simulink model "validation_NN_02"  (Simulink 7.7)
settings: Solver=VariableStepDiscrete  StartTime=0.0  StopTime=100  RelTol=1e-3
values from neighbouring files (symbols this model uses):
  A = [0.9944 -0.1203 -0.4302    [process_model02.m]
  B = [1 0    [process_model02.m]
  C = [1 0 0    [process_model02.m]
  D = zeros(2,2)    [process_model02.m]
  Ts = 0.1    [process_model02.m]
  x0 = [0.01 0.02 0.03]    [process_model02.m]
libraries: neural x21, simulink x6

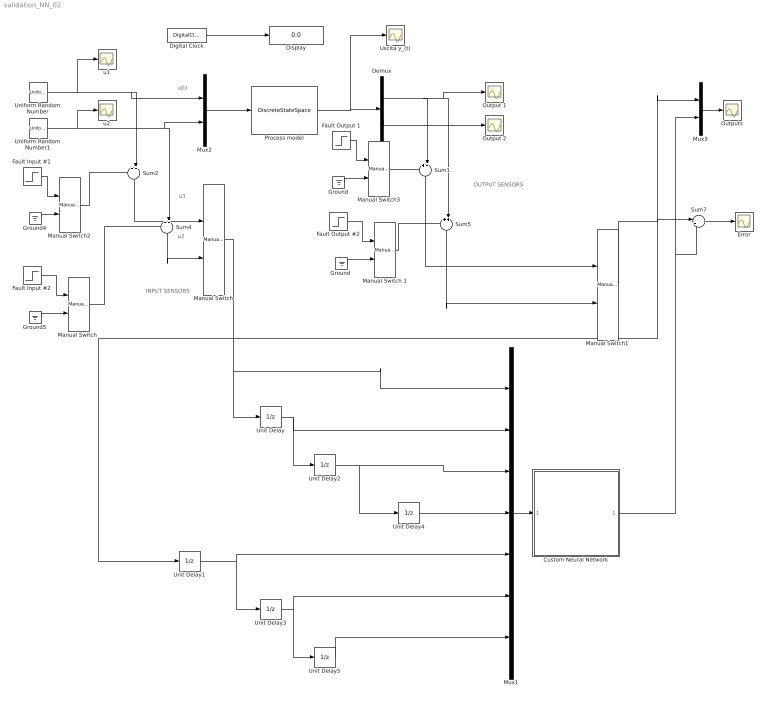
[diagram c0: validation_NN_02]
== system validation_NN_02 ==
  note: u(t)
  note: INPUT SENSORS
  note: OUTPUT SENSORS
  note: u1
  note: u2
  Custom Neural Network : Subsystem
  Demux : Demux  Outputs=2
  Digital Clock : DigitalClock  SampleTime=Ts
  Display : Display
  Error : Scope
  Fault Input #1 : Step  Time=50  After=5  SampleTime=Ts
  Fault Input #2 : Step  Time=50  After=5  SampleTime=Ts
  Fault Output #2 : Step  Time=50  After=5  SampleTime=Ts
  Fault Output 1 : Step  Time=50  After=100  SampleTime=Ts
  Ground : Ground
  "Ground " : Ground
  Ground4 : Ground
  Ground5 : Ground
  Manual Switch : simulink/Signal Routing/Manual Switch  SystemSampleTime=-1  sw=1  action=0  varsize=off
  "Manual Switch " : simulink/Signal Routing/Manual Switch  SystemSampleTime=-1  sw=0  action=0  varsize=off
  Manual Switch 1 : simulink/Signal Routing/Manual Switch  SystemSampleTime=-1  sw=0  action=0  varsize=off
  Manual Switch1 : simulink/Signal Routing/Manual Switch  SystemSampleTime=-1  sw=1  action=0  varsize=off
  Manual Switch2 : simulink/Signal Routing/Manual Switch  SystemSampleTime=-1  sw=0  action=0  varsize=off
  Manual Switch3 : simulink/Signal Routing/Manual Switch  SystemSampleTime=-1  sw=0  action=0  varsize=off
  Mux1 : Mux  Inputs=7
  Mux2 : Mux  Inputs=2
  Mux3 : Mux  Inputs=2
  Output 1 : Scope
  Output 2 : Scope
  Outputs : Scope
  Process model : DiscreteStateSpace  A=A  B=B  C=C  D=D  X0=x0  SampleTime=Ts
  Sum{1..2,4..5} (4 alike) : Sum  Inputs=++|
  Sum7 : Sum  Inputs=|+-
  Uniform Random Number : UniformRandomNumber  Seed=11  SampleTime=Ts
  Uniform Random Number1 : UniformRandomNumber  Minimum=-0.5  Maximum=0.5  Seed=13  SampleTime=Ts
  Unit Delay{,1..5} (6 alike) : UnitDelay  SampleTime=Ts
  Uscita y_(t) : Scope
  u1 : Scope
  u2 : Scope
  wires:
  Digital Clock/1 -> Display/1
  Mux2/1 -> Process model/1
  Uniform Random Number/1 -> u1/1, Mux2/1, Sum2/2
  Process model/1 -> Uscita y_(t)/1, Demux/1
  Uniform Random Number1/1 -> u2/1, Mux2/2, Sum4/2
  Demux/1 -> Output 1/1, Sum5/2, Sum1/2
  Demux/2 -> Output 2/1
  Sum2/1 -> Manual Switch/1
  Sum4/1 -> Manual Switch/2
  Manual Switch/1 -> Unit Delay/1, Mux1/1
  Unit Delay/1 -> Unit Delay2/1, Mux1/2
  Sum1/1 -> Manual Switch1/1
  Sum5/1 -> Manual Switch1/2
  Unit Delay1/1 -> Unit Delay3/1, Mux1/5
  Manual Switch1/1 -> Unit Delay1/1, Sum7/1, Mux3/1
  Sum7/1 -> Error/1
  Unit Delay2/1 -> Unit Delay4/1, Mux1/3
  Unit Delay3/1 -> Unit Delay5/1, Mux1/6
  Unit Delay4/1 -> Mux1/4
  Unit Delay5/1 -> Mux1/7
  Mux3/1 -> Outputs/1
  Custom Neural Network/1(Output) -> Mux3/2, Sum7/2
  Mux1/1 -> Custom Neural Network/1(Input)
  Ground4/1 -> Manual Switch2/2
  Fault Input #1/1 -> Manual Switch2/1
  Fault Input #2/1 -> "Manual Switch "/1
  "Manual Switch "/1 -> Sum4/1
  Manual Switch2/1 -> Sum2/1
  Ground5/1 -> "Manual Switch "/2
  Ground/1 -> Manual Switch3/2
  Fault Output 1/1 -> Manual Switch3/1
  "Ground "/1 -> Manual Switch 1/2
  Fault Output #2/1 -> Manual Switch 1/1
  Manual Switch 1/1 -> Sum5/1
  Manual Switch3/1 -> Sum1/1

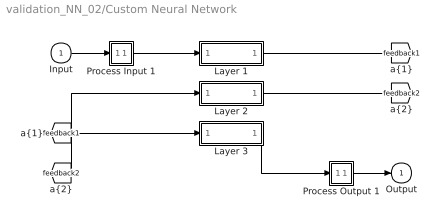
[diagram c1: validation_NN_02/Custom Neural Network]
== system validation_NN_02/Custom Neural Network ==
  Input : Inport  PortDimensions=7
  Layer 1 : Subsystem
  Layer 2 : Subsystem
  Layer 3 : Subsystem
  Process Input 1 : Subsystem
  Process Output 1 : Subsystem
  Output : Outport  InitialOutput=0
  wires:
  Input/1 -> Process Input 1/1(x)
  Process Output 1/1(y) -> Output/1
  Process Input 1/1(p) -> Layer 1/1("p{1}")
  Layer 1/1("a{1}") -> [feedback1]
  [feedback1] -> Layer 2/1("a{1} ")
  Layer 2/1("a{2}") -> [feedback2]
  [feedback2] -> Layer 3/1("a{2} ")
  Layer 3/1("a{3}") -> Process Output 1/1(a)

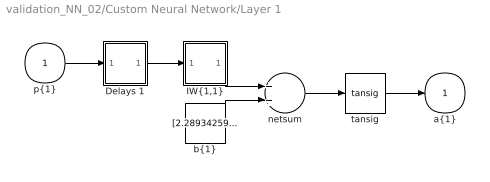
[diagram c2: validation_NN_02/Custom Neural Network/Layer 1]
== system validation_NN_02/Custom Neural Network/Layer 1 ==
  "p{1}" : Inport  PortDimensions=7
  Delays 1 : Subsystem
  "IW{1,1}" : Subsystem
  "b{1}" : Constant  Value=[2.2893425931778344;1.1932961118015271;0.26357406309628256;1.4693944586922609]
  netsum : Sum  Inputs=2
  tansig : neural/Transfer Functions/tansig  SystemSampleTime=-1
  "a{1}" : Outport  InitialOutput=[0;0;0;0]
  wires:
  "p{1}"/1 -> Delays 1/1("p{1}")
  Delays 1/1("pd{1,1}") -> "IW{1,1}"/1("pd{1,1}")
  "IW{1,1}"/1("iz{1,1}") -> netsum/1
  "b{1}"/1 -> netsum/2
  netsum/1 -> tansig/1
  tansig/1 -> "a{1}"/1

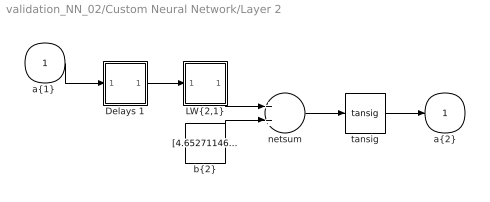
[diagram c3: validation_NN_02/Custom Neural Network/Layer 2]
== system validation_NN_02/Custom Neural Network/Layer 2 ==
  "a{1} " : Inport  PortDimensions=4
  Delays 1 : Subsystem
  "LW{2,1}" : Subsystem
  "b{2}" : Constant  Value=[4.6527114652012163;-0.20165441708959697;5.1786637975381806;-0.85155381578495404;2.066754727326872;1.0542387931417163;2.3683712400664416;-0.63100835699891689]
  netsum : Sum  Inputs=2
  tansig : neural/Transfer Functions/tansig  SystemSampleTime=-1
  "a{2}" : Outport  InitialOutput=[0;0;0;0;0;0;0;0]
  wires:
  "a{1} "/1 -> Delays 1/1("p{2}")
  Delays 1/1("pd{2,1}") -> "LW{2,1}"/1("ad{2,1}")
  "LW{2,1}"/1("lz{2,1}") -> netsum/1
  "b{2}"/1 -> netsum/2
  netsum/1 -> tansig/1
  tansig/1 -> "a{2}"/1

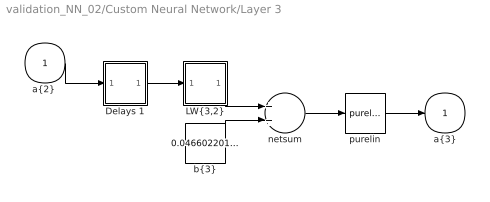
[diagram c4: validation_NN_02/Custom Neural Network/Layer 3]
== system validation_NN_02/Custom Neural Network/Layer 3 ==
  "a{2} " : Inport  PortDimensions=8
  Delays 1 : Subsystem
  "LW{3,2}" : Subsystem
  "b{3}" : Constant  Value=0.046602201697887827
  netsum : Sum  Inputs=2
  purelin : neural/Transfer Functions/purelin  SystemSampleTime=-1
  "a{3}" : Outport  InitialOutput=0
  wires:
  "a{2} "/1 -> Delays 1/1("p{3}")
  Delays 1/1("pd{3,2}") -> "LW{3,2}"/1("ad{3,2}")
  "LW{3,2}"/1("lz{3,2}") -> netsum/1
  "b{3}"/1 -> netsum/2
  netsum/1 -> purelin/1
  purelin/1 -> "a{3}"/1

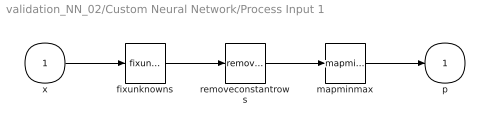
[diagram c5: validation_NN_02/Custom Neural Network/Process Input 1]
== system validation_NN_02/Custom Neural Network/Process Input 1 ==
  x : Inport  PortDimensions=7
  fixunknowns : neural/Processing Functions/fixunknowns  SystemSampleTime=-1  inputSize=7  indices=[1 2 3 4 5 6 7]
  mapminmax : neural/Processing Functions/mapminmax  SystemSampleTime=-1  xmin=[-1.137661454327592;-1.1106929140419901;-1.121216738180955;-1.1470725250976375;-31.095443858794159;-31.404321949219387;-30.957687527471332]  xmax=[1.1540492640826692;1.122893357889289;1.1111953057620241;1.1421296989998391;32.607744268199028;33.039723432629302;33.345757904804152]  ymin=-1  ymax=1
  removeconstantrows : neural/Processing Functions/removeconstantrows  SystemSampleTime=-1  inputSize=7  keep=[1 2 3 4 5 6 7]
  p : Outport  PortDimensions=7
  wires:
  x/1 -> fixunknowns/1
  fixunknowns/1 -> removeconstantrows/1
  removeconstantrows/1 -> mapminmax/1
  mapminmax/1 -> p/1

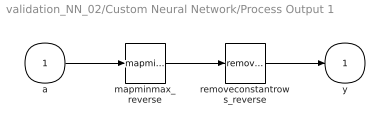
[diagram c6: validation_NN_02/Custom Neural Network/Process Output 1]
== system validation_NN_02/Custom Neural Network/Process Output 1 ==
  a : Inport  PortDimensions=1
  mapminmax_reverse : neural/Processing Functions/mapminmax_reverse  SystemSampleTime=-1  xmin=-31.173256733227603  xmax=32.664397268400201  ymin=-1  ymax=1
  removeconstantrows_reverse : neural/Processing Functions/removeconstantrows_reverse  SystemSampleTime=-1  inputSize=1  constants=zeros(0,1)  rearrange=1
  y : Outport  PortDimensions=1
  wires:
  a/1 -> mapminmax_reverse/1
  mapminmax_reverse/1 -> removeconstantrows_reverse/1
  removeconstantrows_reverse/1 -> y/1

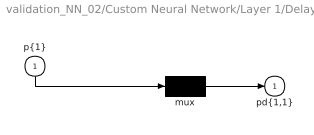
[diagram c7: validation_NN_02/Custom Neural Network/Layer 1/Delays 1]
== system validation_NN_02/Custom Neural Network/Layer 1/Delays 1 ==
  "p{1}" : Inport  PortDimensions=7
  mux : Mux  Inputs=1
  "pd{1,1}" : Outport
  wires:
  "p{1}"/1 -> mux/1
  mux/1 -> "pd{1,1}"/1

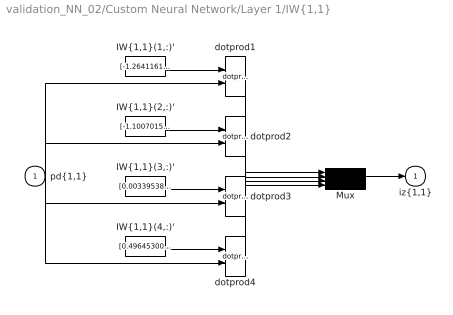
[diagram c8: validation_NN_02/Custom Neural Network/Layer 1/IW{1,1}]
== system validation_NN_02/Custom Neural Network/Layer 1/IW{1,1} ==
  "pd{1,1}" : Inport  PortDimensions=7
  "IW{1,1}(1,:)'" : Constant  Value=[-1.2641161299487504;0.0997384285530524;1.2284773037160353;0.7475180490745561;-0.7399779544886097;0.39704162573921498;1.3750797954397804]
  "IW{1,1}(2,:)'" : Constant  Value=[-1.1007015532539755;-0.37448883843292025;-0.11491510471219206;0.74396610481719905;-1.6153284054239792;-0.62048648970817799;-0.57032641425918018]
  "IW{1,1}(3,:)'" : Constant  Value=[0.003395389549716609;0.0046069654091452856;-0.0013782220466399151;-0.0028529495459147058;0.094167514180012443;0.040073664339456375;-0.014230724676680765]
  "IW{1,1}(4,:)'" : Constant  Value=[0.49645300652299523;0.063835313117828529;-0.33573042533020231;-0.37637796015789859;0.41313196516445566;0.046904745501174454;-0.74678156912160532]
  Mux : Mux
  dotprod{1..4} (4 alike) : neural/Weight Functions/dotprod  SystemSampleTime=-1
  "iz{1,1}" : Outport
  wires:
  "IW{1,1}(1,:)'"/1 -> dotprod1/1
  "pd{1,1}"/1 -> dotprod1/2, dotprod2/2, dotprod3/2, dotprod4/2
  dotprod1/1 -> Mux/1
  "IW{1,1}(2,:)'"/1 -> dotprod2/1
  dotprod2/1 -> Mux/2
  "IW{1,1}(3,:)'"/1 -> dotprod3/1
  dotprod3/1 -> Mux/3
  "IW{1,1}(4,:)'"/1 -> dotprod4/1
  dotprod4/1 -> Mux/4
  Mux/1 -> "iz{1,1}"/1

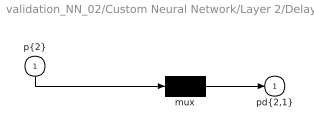
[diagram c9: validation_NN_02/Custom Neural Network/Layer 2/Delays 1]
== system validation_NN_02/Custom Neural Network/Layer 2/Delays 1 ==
  "p{2}" : Inport  PortDimensions=4
  mux : Mux  Inputs=1
  "pd{2,1}" : Outport
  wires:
  "p{2}"/1 -> mux/1
  mux/1 -> "pd{2,1}"/1

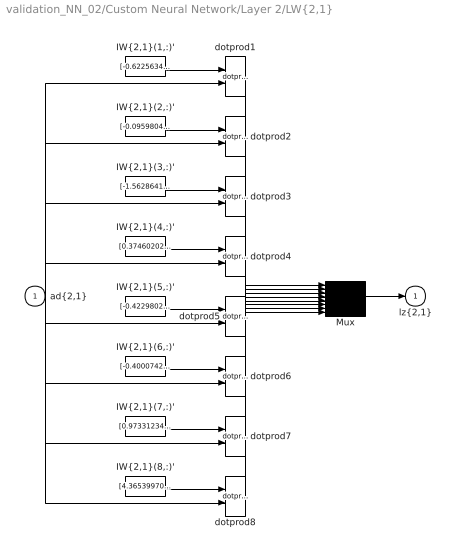
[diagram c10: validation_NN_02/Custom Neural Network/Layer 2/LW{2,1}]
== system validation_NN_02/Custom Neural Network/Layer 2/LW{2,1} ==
  "ad{2,1}" : Inport  PortDimensions=4
  "IW{2,1}(1,:)'" : Constant  Value=[-0.6225634803186495;0.056019752416234123;3.8317385529771952;-3.9152656035632489]
  "IW{2,1}(2,:)'" : Constant  Value=[-0.095980493880186951;-0.020787011272775074;2.015485309832703;-0.50241908048017825]
  "IW{2,1}(3,:)'" : Constant  Value=[-1.5628641767532132;2.7100511580180426;-4.4478678297847054;-2.1967938993031892]
  "IW{2,1}(4,:)'" : Constant  Value=[0.37460202059424275;0.28802119681258126;-0.69407467364564313;0.84657587195097128]
  "IW{2,1}(5,:)'" : Constant  Value=[-0.42298025230215686;-0.13564419327262969;-2.3017326521045662;-1.2375246405668017]
  "IW{2,1}(6,:)'" : Constant  Value=[-0.40007420276913397;-0.26246678030892368;-0.61107355074929448;0.34951665213791755]
  "IW{2,1}(7,:)'" : Constant  Value=[0.97331234014830192;2.8732917125244044;-0.99904470595644546;-2.6441388017316205]
  "IW{2,1}(8,:)'" : Constant  Value=[4.3653997044932895;-0.22618936910412749;0.081171926245456924;-0.81857236329042427]
  Mux : Mux  Inputs=8
  dotprod{1..8} (8 alike) : neural/Weight Functions/dotprod  SystemSampleTime=-1
  "lz{2,1}" : Outport
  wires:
  "IW{2,1}(1,:)'"/1 -> dotprod1/1
  "ad{2,1}"/1 -> dotprod1/2, dotprod2/2, dotprod3/2, dotprod4/2, dotprod5/2, dotprod6/2, dotprod7/2, dotprod8/2
  dotprod1/1 -> Mux/1
  "IW{2,1}(2,:)'"/1 -> dotprod2/1
  dotprod2/1 -> Mux/2
  "IW{2,1}(3,:)'"/1 -> dotprod3/1
  dotprod3/1 -> Mux/3
  "IW{2,1}(4,:)'"/1 -> dotprod4/1
  dotprod4/1 -> Mux/4
  "IW{2,1}(5,:)'"/1 -> dotprod5/1
  dotprod5/1 -> Mux/5
  "IW{2,1}(6,:)'"/1 -> dotprod6/1
  dotprod6/1 -> Mux/6
  "IW{2,1}(7,:)'"/1 -> dotprod7/1
  dotprod7/1 -> Mux/7
  "IW{2,1}(8,:)'"/1 -> dotprod8/1
  dotprod8/1 -> Mux/8
  Mux/1 -> "lz{2,1}"/1

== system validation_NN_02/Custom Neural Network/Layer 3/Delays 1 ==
  "p{3}" : Inport  PortDimensions=8
  mux : Mux  Inputs=1
  "pd{3,2}" : Outport
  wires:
  "p{3}"/1 -> mux/1
  mux/1 -> "pd{3,2}"/1

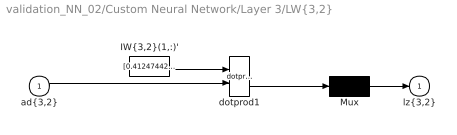
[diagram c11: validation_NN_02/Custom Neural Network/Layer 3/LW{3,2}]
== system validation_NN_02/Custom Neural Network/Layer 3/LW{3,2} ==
  "ad{3,2}" : Inport  PortDimensions=8
  "IW{3,2}(1,:)'" : Constant  Value=[0.41247442918091326;3.0793533739304646;0.0098486080117294334;-0.13070822636330165;-1.1978322964783754;0.35806407360085035;-0.019173693485791565;-0.020610836955466508]
  Mux : Mux  Inputs=1
  dotprod1 : neural/Weight Functions/dotprod  SystemSampleTime=-1
  "lz{3,2}" : Outport
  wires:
  "IW{3,2}(1,:)'"/1 -> dotprod1/1
  "ad{3,2}"/1 -> dotprod1/2
  dotprod1/1 -> Mux/1
  Mux/1 -> "lz{3,2}"/1
